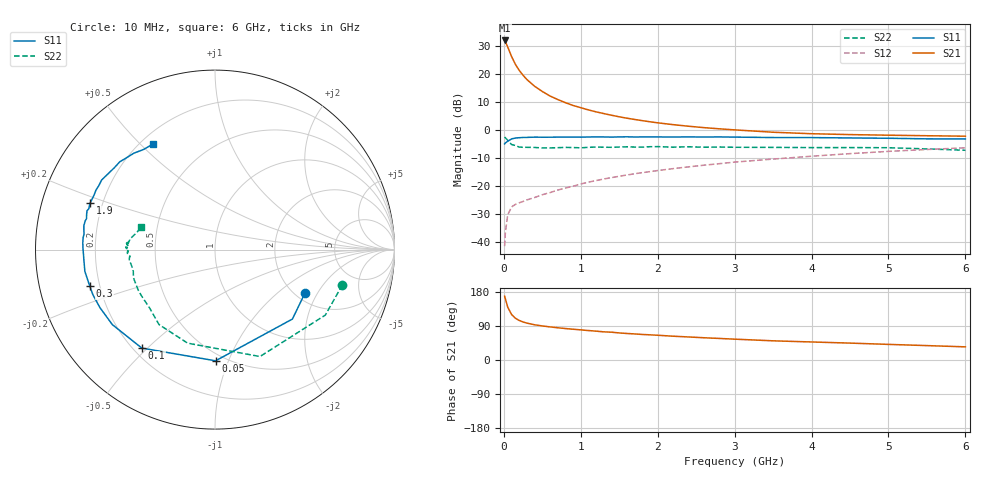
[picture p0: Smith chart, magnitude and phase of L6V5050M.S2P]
!  INFINEON TECHNOLOGIES Small Signal Semiconductors
! BFR380L3 , Si-NPN RF-Transistor in TSLP-3-1
!  Vce=0.5 V,  Ic=50 mA
! Common Emitter S-Parameters:  07. March 2005
#  GHz  S  MA  R  50
! f  S11  S21  S12  S22
! GHz  Mag  Ang  Mag  Ang  Mag  Ang  Mag  Ang
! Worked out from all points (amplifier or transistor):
!   36 points, 10 MHz to 6 GHz, reference 50 ohm
!   highest |S21| = 31.9 dB at 10 MHz (marker M1)
!   |S21| within 3 dB of that: start of sweep to 60.2 MHz
!   unconditionally stable (mu >= 1): 744.4 MHz to end of sweep
!   at 250 MHz: K = 0.59, MSG = 22.5 dB, |S12| = -25.6 dB
!   at 1.4 GHz: K = 1.12, MAG = 9.1 dB, |S12| = -17.1 dB
!   at 6 GHz: K = 1.05, MAG = 0.7 dB, |S12| = -6.5 dB
!   S11 on the Smith chart (normalised r, x): 10 MHz: 2.24, -1.58; 50 MHz: 0.45, -0.90; 100 MHz: 0.23, -0.48; 300 MHz: 0.16, -0.14; 1.9 GHz: 0.15, +0.18; 6 GHz: 0.25, +0.55
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0.01  0.5567 -25.8  39.16 168.3  0.0083 70.4  0.7365 -15.5
0.02  0.5794 -41.9  37.33 161.3  0.0146 67.7  0.7148 -30.7
0.05  0.6196 -89.7  30.03 139.7  0.0299 53.7  0.6463 -67.2
0.1  0.6835 -126.6  20.3 120.2  0.0417 41.0  0.5431 -106.3
0.15  0.7084 -143.8  14.71 110.2  0.0462 37.4  0.5212 -126.8
0.2  0.7179 -153.2  11.44 104.4  0.0494 38.3  0.4887 -138.1
0.25  0.7253 -159.7  9.356 100.3  0.0522 38.3  0.4838 -147.7
0.3  0.7268 -163.8  7.846 97.4  0.0556 40.5  0.4836 -152.3
0.4  0.7351 -170.5  5.959 92.9  0.0614 43.8  0.4808 -161.0
0.5  0.7328 -174.8  4.803 89.9  0.0689 47.6  0.4709 -165.2
0.6  0.7332 -177.8  3.991 87.3  0.0751 50.4  0.4718 -168.0
0.7  0.7354 179.8  3.454 85.1  0.0833 53.2  0.4764 -170.9
0.8  0.7376 177.0  3.036 83.0  0.0905 55.1  0.4819 -172.7
0.9  0.7377 174.7  2.703 81.2  0.0977 56.5  0.4788 -174.7
1.1  0.7391 171.4  2.25 77.7  0.1155 58.6  0.4837 -176.0
1.5  0.7416 164.7  1.696 71.4  0.1471 60.6  0.4894 -179.2
1.9  0.742 159.6  1.382 66.4  0.1779 61.0  0.4958 178.8
2.2  0.7391 155.7  1.229 62.8  0.2013 60.8  0.486 177.7
3.5  0.7228 140.8  0.899 50.6  0.298 57.5  0.482 174.6
4.5  0.711 134.1  0.816 44.6  0.3729 54.1  0.4786 173.2
5.5  0.685 125.4  0.779 38.0  0.4424 48.7  0.4531 169.0
6  0.6819 120.3  0.764 34.7  0.4741 46.0  0.4281 163.2
